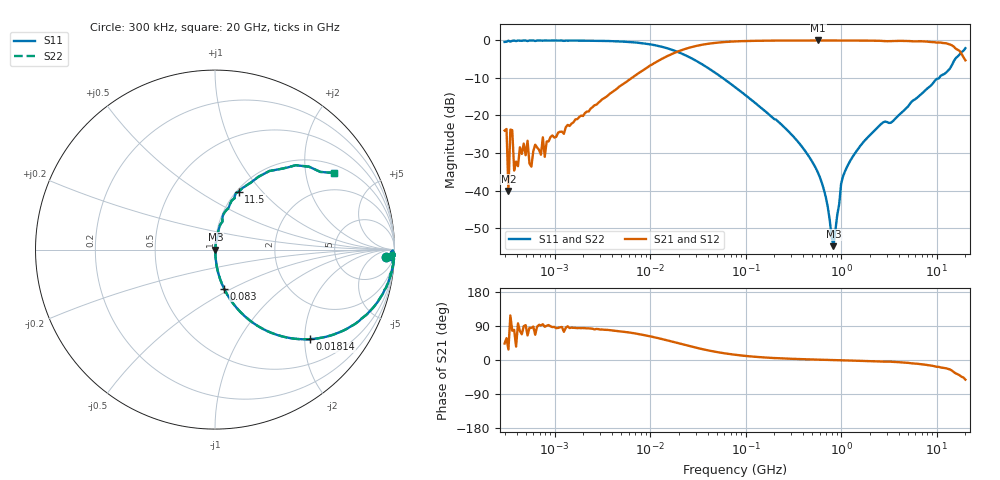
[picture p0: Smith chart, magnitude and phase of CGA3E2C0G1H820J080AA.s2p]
! S-parameter Generated by TDK Corporation
! Copyright(C) 2015 TDK Corporation.
! All Rights Reserved.
! TDK P/N: CGA3E2C0G1H820J080AA (Multilayer Ceramic Chip Capacitors)
! Property: C=82pF
! Size(LxWxT): 1.6x0.8x0.8mm, 0.063x0.031x0.031inches
! Model Type: s2p (Touchstone File Format Version 1.0)
! Frequency: DC=Yes Start=0.3MHz Stop=20000MHz 243points Log-sweep
! Note:
! Model Generated on Jun. 23, 2015
! Hash(MD5):
! Port Assignments:
!  1 ---| |--- 2
! Applicable Conditions:
!  Temperature = 25 degC
!  DC Bias Voltage = 0 V
!  Small Signal Operation
! Terms and conditions regarding TDK Simulation Models
! (1)This simulation model is being provided solely for informational purposes. Please refer to the specifications of the products in terms of detailed characteristics of such products.
! (2)In no event shall TDK Corporation of any of its subsidiaries be liable for any loss or damage arising, directly or indirectly,
!  From any information contained in this simulation model, including, but not limited to loss or damages arising from any inaccuracies, omissions or errors in connection with such information.
! (3)Any and all copyrights on this simulation model are owned by TDK Corporation.
!  Duplication or redistribution of this simulation model without prior written permission from TDK Corporation is prohibited.
! (4)This simulation model is subject to any modification or change without any prior notice.
! (5)Neither TDK Corporation nor any of its subsidiaries shall make any warranty, express or implied,
!  Including but not limited to the correctness, implied warranties of merchantability and fitness for a particular purpose with respect to this simulation models.
! (6)The use of this simulation model shall be deemed to have consented to the terms and conditions hereof.
# MHz S MA R 50
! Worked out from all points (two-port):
!   242 points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, 300 kHz to 20 GHz, reference 50 ohm
!   highest |S21| = -0.01 dB at 575.2 MHz (marker M1); lowest = -40.1 dB at 329 kHz (marker M2)
!   |S21| within 3 dB of the highest: 19.28 MHz to 17.64 GHz (17.62 GHz wide, 200 % of centre)
!   lowest |S11| = -54.8 dB at 831.6 MHz (marker M3), VSWR 1.00, Z = 50.2 + j0.03 ohm
!   |S11| at or under -10 dB: 57.5 MHz to 10.61 GHz (10.55 GHz wide, 198 % of centre)
!   |S22| runs from -54.8 to 0.0 dB; largest |S21 - S12| = 0
!   S11 on the Smith chart (normalised r, x): 300 kHz: 22, -22; 18.14 MHz: 1.00, -2.12; 83 MHz: 1.00, -0.46; 11.5 GHz: 1.02, +0.75; 20 GHz: 1.28, +2.89
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0.3  0.9552 -2.6  0.06301 43.4  0.06301 43.4  0.9552 -2.6
0.3141503  0.9622 -2.8  0.06607 57.7  0.06607 57.7  0.9622 -2.8
0.328968  0.9912 -0.3  0.0099 27.5  0.0099 27.5  0.9912 -0.3
0.3444847  0.9652 -3.4  0.06475 117.5  0.06475 117.5  0.9652 -3.4
0.3607332  0.9877 -3.4  0.06371 77.3  0.06371 77.3  0.9877 -3.4
0.3777482  0.9968 -0.9  0.01844 79.6  0.01844 79.6  0.9968 -0.9
0.4756456  0.9978 -2.4  0.04223 89.3  0.04223 89.3  0.9978 -2.4
0.5719372  0.9984 -1.2  0.02078 84.9  0.02078 84.9  0.9984 -1.2
0.6271635  0.983 -2.0  0.04079 66.7  0.04079 66.7  0.983 -2.0
0.7896995  0.9992 -1.6  0.02812 87.7  0.02812 87.7  0.9992 -1.6
1.985118  0.9951 -5.7  0.09851 84.3  0.09851 84.3  0.9951 -5.7
12.54397  0.8376 -33.1  0.5457 56.9  0.5457 56.9  0.8376 -33.1
18.13697  0.728 -43.3  0.6853 46.7  0.6853 46.7  0.728 -43.3
79.26541  0.2337 -76.3  0.9717 13.5  0.9717 13.5  0.2337 -76.3
83.00418  0.2235 -76.9  0.9741 12.9  0.9741 12.9  0.2235 -76.9
500.8786  0.02394 -85.3  0.9983 1.4  0.9983 1.4  0.02394 -85.3
575.15  0.01705 -84.2  0.9984 1.0  0.9984 1.0  0.01705 -84.2
831.5931  0.001813 9.5  0.9982 -0.0  0.9982 -0.0  0.001813 9.5
1096.499  0.01795 81.0  0.9973 -1.0  0.9973 -1.0  0.01795 81.0
3165.055  0.07946 72.2  0.9787 -4.4  0.9787 -4.4  0.07946 72.2
11503.64  0.3481 67.8  0.9263 -20.4  0.9263 -20.4  0.3481 67.8
20000  0.789 32.7  0.5434 -51.7  0.5434 -51.7  0.789 32.7
